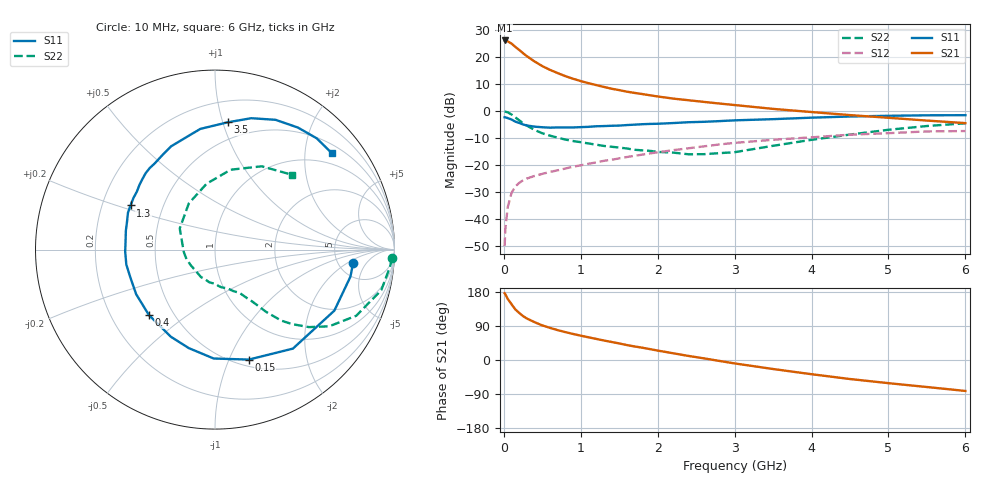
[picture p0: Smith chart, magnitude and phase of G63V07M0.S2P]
! SIEMENS Small Signal Semiconductors
! BFG193
! Si NPN RF Bipolar Junction Transistor in SOT223
! VCE = 3 V  IC = 7 mA
! Common Emitter S-Parameters:  August  1996
# GHz  S  MA  R  50
!  f  S11  S21  S12  S22
! GHz  MAG  ANG  MAG  ANG  MAG  ANG  MAG  ANG
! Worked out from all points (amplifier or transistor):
!   36 points, 10 MHz to 6 GHz, reference 50 ohm
!   highest |S21| = 26.2 dB at 10 MHz (marker M1)
!   |S21| within 3 dB of that: start of sweep to 177.2 MHz
!   unconditionally stable (mu >= 1): 998.2 MHz to 2.601 GHz
!   at 250 MHz: K = 0.43, MSG = 23.5 dB, |S12| = -25.5 dB
!   at 1.4 GHz: K = 1.08, MAG = 11.4 dB, |S12| = -18.0 dB
!   at 6 GHz: K = 0.88, MSG = 1.5 dB, |S12| = -7.3 dB
!   S11 on the Smith chart (normalised r, x): 10 MHz: 6.90, -2.50; 150 MHz: 0.57, -1.19; 400 MHz: 0.36, -0.36; 1.3 GHz: 0.32, +0.22; 3.5 GHz: 0.36, +1.04; 6 GHz: 0.70, +2.63
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0.01  0.7732 -5.4  20.3 176.2  0.0032 92.9  0.9876 -2.8
0.02  0.7696 -11.3  20.25 173.2  0.0067 82.2  0.9798 -5.6
0.05  0.7468 -27.1  19.56 161.4  0.0167 77.2  0.9537 -13.7
0.1  0.7019 -51.8  17.76 147.2  0.0309 66.5  0.869 -25.1
0.15  0.6411 -72.9  15.43 133.4  0.0407 57.6  0.7663 -33.9
0.2  0.6069 -90.7  13.55 124.1  0.0474 52.8  0.6789 -39.5
0.25  0.5679 -104.9  11.81 115.8  0.0528 48.9  0.5979 -44.0
0.3  0.5444 -116.8  10.38 109.4  0.057 47.0  0.5407 -47.0
0.4  0.5181 -135.3  8.29 99.8  0.0636 44.3  0.4495 -50.6
0.5  0.5047 -150.5  6.81 91.3  0.0694 43.2  0.391 -52.7
0.6  0.4964 -161.7  5.808 84.8  0.0755 43.8  0.3531 -54.5
0.7  0.5011 -170.4  5.057 78.8  0.0808 43.8  0.3238 -56.6
0.9  0.5005 174.6  3.98 68.7  0.094 43.8  0.2809 -60.0
1.1  0.5139 162.6  3.296 59.9  0.1065 43.7  0.2535 -66.0
1.3  0.5311 152.4  2.811 51.5  0.1208 43.0  0.2281 -71.6
1.7  0.5639 135.8  2.178 35.7  0.1497 39.7  0.1937 -88.0
2.2  0.6036 118.8  1.71 17.8  0.1903 32.4  0.1717 -117.1
2.8  0.6554 101.8  1.387 -2.4  0.2427 21.9  0.1676 -161.4
3.5  0.7127 84.3  1.103 -23.8  0.2963 6.4  0.2292 149.0
4.5  0.7979 65.0  0.847 -50.2  0.3678 -13.7  0.3698 97.3
5.5  0.8399 47.6  0.671 -71.3  0.4231 -38.4  0.5322 60.7
6  0.8443 39.4  0.602 -81.7  0.4296 -52.7  0.5974 44.3
